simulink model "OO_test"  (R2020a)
settings: Solver=ode45  StartTime=0.0  StopTime=2000  RelTol=1e-3  EnableMultiTasking=on
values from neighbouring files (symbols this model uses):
  Ts = 0.2    [init_model.m]
libraries: ctrlSharedLib x1

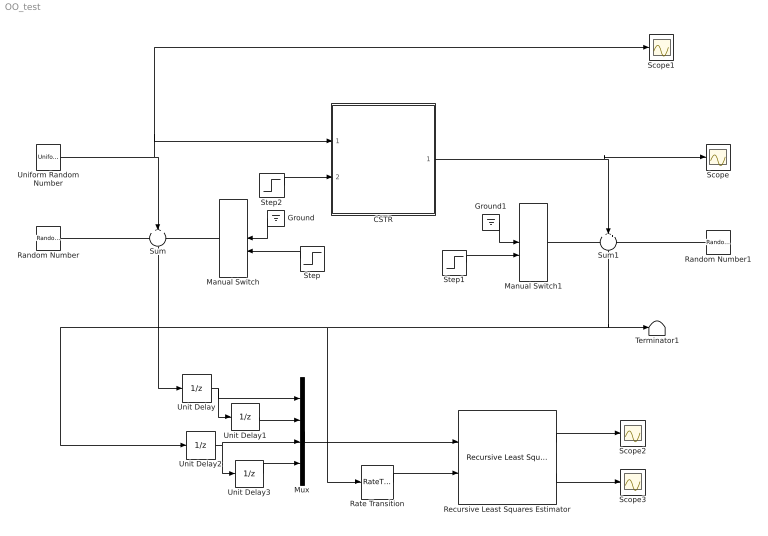
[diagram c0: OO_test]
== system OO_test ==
  CSTR : Subsystem
  Ground : Ground
  Ground1 : Ground
  Manual Switch : ManualSwitch
  Manual Switch1 : ManualSwitch
  Mux : Mux
  Random Number : RandomNumber  Variance=0.0001  Seed=1  SampleTime=Ts
  Random Number1 : RandomNumber  Variance=0.0005  Seed=2  SampleTime=Ts
  Rate Transition : RateTransition
  Recursive Least Squares Estimator : ctrlSharedLib/Recursive Least Squares Estimator  InitialEstimateSource=None  InitialParameterData=4  P0=1e4  InitialRegressors=0  InitialOutputs=0  History=Infinite  WindowLength=200  EstimationMethod=Forgetting Factor  AdaptationParameter=1  HasTimeVaryingAdaptationParameter=off  NormalizationBias=eps  OutputError=on  OutputP=off  AddEnablePort=off  InputProcessing=Sample-based  Ts=Ts
  Scope{,1..3} (4 alike) : Scope
  Step : Step  Time=900  SampleTime=0
  Step1 : Step  Time=1000  After=10  SampleTime=0
  Step2 : Step  Time=1000  SampleTime=0
  Sum : Sum  Inputs=+++  SaturateOnIntegerOverflow=on
  Sum1 : Sum  Inputs=+++  SaturateOnIntegerOverflow=on
  Terminator1 : Terminator
  Uniform Random Number : UniformRandomNumber  Minimum=0  Maximum=4  SampleTime=20
  Unit Delay{,1..3} (4 alike) : UnitDelay  SampleTime=Ts  HasFrameUpgradeWarning=on
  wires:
  Uniform Random Number/1 -> CSTR/1(w), Scope1/1, Sum/2
  Random Number/1 -> Sum/1
  Manual Switch/1 -> Sum/3
  Sum/1 -> Unit Delay/1
  Ground/1 -> Manual Switch/1
  Step/1 -> Manual Switch/2
  Ground1/1 -> Manual Switch1/1
  Step1/1 -> Manual Switch1/2
  CSTR/1(Cb) -> Scope/1, Sum1/2
  Sum1/1 -> Rate Transition/1, Unit Delay2/1, Terminator1/1
  Manual Switch1/1 -> Sum1/1
  Random Number1/1 -> Sum1/3
  Step2/1 -> CSTR/2(f)
  Unit Delay/1 -> Unit Delay1/1, Mux/1
  Unit Delay1/1 -> Mux/2
  Unit Delay2/1 -> Mux/3, Unit Delay3/1
  Unit Delay3/1 -> Mux/4
  Mux/1 -> Recursive Least Squares Estimator/1
  Rate Transition/1 -> Recursive Least Squares Estimator/2
  Recursive Least Squares Estimator/1 -> Scope2/1
  Recursive Least Squares Estimator/2 -> Scope3/1

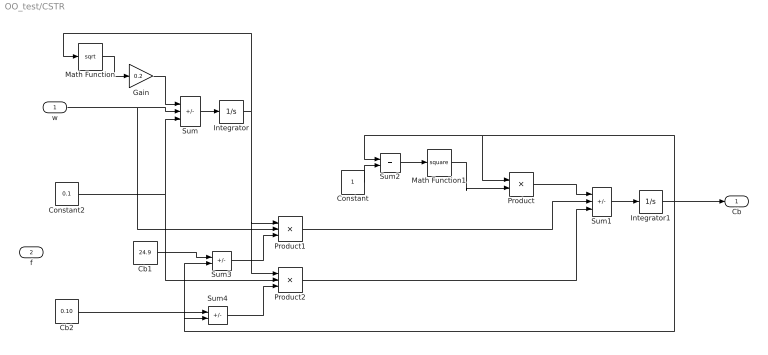
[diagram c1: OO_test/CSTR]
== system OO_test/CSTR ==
  w : Inport
  f : Inport  Port=2
  Cb1 : Constant  Value=24.9
  Cb2 : Constant  Value=0.10
  Constant : Constant
  Constant2 : Constant  Value=0.1
  Gain : Gain  Gain=0.2  SaturateOnIntegerOverflow=on
  Integrator : Integrator  InitialCondition=30  LimitOutput=on  LowerSaturationLimit=1
  Integrator1 : Integrator  InitialCondition=22
  Math Function : Math  Operator=sqrt
  Math Function1 : Math  Operator=square
  Product : Product  Inputs=*/  SaturateOnIntegerOverflow=on
  Product1 : Product  Inputs=/**  SaturateOnIntegerOverflow=on
  Product2 : Product  Inputs=/**  SaturateOnIntegerOverflow=on
  Sum : Sum  Inputs=-++  SaturateOnIntegerOverflow=on
  Sum1 : Sum  Inputs=-++  SaturateOnIntegerOverflow=on
  Sum2 : Sum  SaturateOnIntegerOverflow=on
  Sum3 : Sum  Inputs=+-  SaturateOnIntegerOverflow=on
  Sum4 : Sum  Inputs=+-  SaturateOnIntegerOverflow=on
  Cb : Outport
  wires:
  Sum/1 -> Integrator/1
  Gain/1 -> Sum/1
  Math Function/1 -> Gain/1
  Integrator/1 -> Math Function/1, Product1/1, Product2/1
  Cb1/1 -> Sum3/1
  Cb2/1 -> Sum4/1
  Sum3/1 -> Product1/3
  Sum4/1 -> Product2/3
  Constant/1 -> Sum2/2
  Sum2/1 -> Math Function1/1
  Sum1/1 -> Integrator1/1
  Math Function1/1 -> Product/2
  Product/1 -> Sum1/1
  Product1/1 -> Sum1/2
  Product2/1 -> Sum1/3
  w/1 -> Sum/2, Product1/2
  Constant2/1 -> Sum/3, Product2/2
  Integrator1/1 -> Sum3/2, Sum4/2, Sum2/1, Product/1, Cb/1
